[IBIS VER]   4.1
[File Name]   f29h85xpts.ibs
[File Rev]   1.0
[Date]   May 06, 2024
[Source]   File originated at Texas Instruments
[Copyright]   (c) 2012, Texas Instruments Inc.
[Component]   f29h85xpts
[Manufacturer]  Texas Instruments
[Package]
| Variable   Typ   Min   Max
R_pkg   2.65E-01   1.10E-01   3.57E-01
L_pkg   7.29E-09   5.43E-09   8.54E-09
C_pkg   1.07E-13   7.65E-14   2.05E-13
[Pin]   signal_name   model_name   R_pin   L_pin   C_pin
1   GPIO15   BQ33100HYPBFZ_PMB_5FS_LC_7LM   2.94E-01   8.32E-09   2.03E-13
2   GPIO16   BCF33100DSHYPBFZ_USF_7LM   2.97E-01   8.27E-09   1.00E-13
3   VDDIO   NC   2.90E-01   8.13E-09   9.86E-14
4   GPIO17   BCF33100DSHYPBFZ_USF_7LM   2.88E-01   8.03E-09   9.72E-14
5   GPIO19   BCF33100DSHYPBFZ_USF_7LM   2.82E-01   7.90E-09   9.58E-14
6   GPIO20   BCF33100DSHYPBFZ_USF_7LM   2.77E-01   7.78E-09   9.44E-14
7   GPIO21   BCF33100DSHYPBFZ_USF_7LM   2.72E-01   7.66E-09   9.30E-14
8   VDD   NC   1.59E-01   6.53E-09   9.39E-14
9   GPIO34   BCF33100DSHYPBFZ_USF_7LM   2.96E-01   7.73E-09   9.06E-14
10   GPIO35   BCF33100DSHYPBFZ_USF_7LM   2.90E-01   7.59E-09   8.92E-14
11   VDD   NC   1.75E-01   6.46E-09   9.05E-14
12   VDDIO   NC   3.57E-01   8.06E-09   8.71E-14
13   GPIO18   BQ33100HYPBFZ_PMB_5FS_LC_7LM   3.47E-01   7.89E-09   8.56E-14
14   GPIO22   BQ33100HYPBFZ_PMB_5FS_LC_7LM   3.44E-01   7.80E-09   8.43E-14
15   B11,GPIO235   BCF33100DSHYPBFZ_USF_7LM   3.42E-01   7.70E-09   8.29E-14
16   B10,GPIO234   BCF33100DSHYPBFZ_USF_7LM   3.33E-01   7.54E-09   8.15E-14
17   A11,GPIO229   BCF33100DSHYPBFZ_USF_7LM   3.24E-01   7.38E-09   8.01E-14
18   A10,GPIO228   BCF33100DSHYPBFZ_USF_7LM   3.16E-01   7.23E-09   7.86E-14
19   B9,GPIO233   BCF33100DSHYPBFZ_USF_7LM   3.08E-01   7.08E-09   7.72E-14
20   B8,GPIO232   BCF33100DSHYPBFZ_USF_7LM   3.01E-01   6.94E-09   2.04E-13
21   A9,GPIO227   BCF33100DSHYPBFZ_USF_7LM   2.95E-01   6.80E-09   2.00E-13
22   A8,GPIO226   BCF33100DSHYPBFZ_USF_7LM   2.89E-01   6.68E-09   1.96E-13
23   B7/E27,GPIO231   BCF33100DSHYPBFZ_USF_7LM   2.88E-01   6.66E-09   1.96E-13
24   B6/E26,GPIO230   BCF33100DSHYPBFZ_USF_7LM   2.82E-01   6.69E-09   2.00E-13
25   A7/E25,GPIO225   BCF33100DSHYPBFZ_USF_7LM   2.77E-01   6.72E-09   2.03E-13
26   A6/E24,GPIO224   BCF33100DSHYPBFZ_USF_7LM   2.73E-01   6.75E-09   7.69E-14
27   VDDA   NC   1.63E-01   5.81E-09   8.07E-14
28   VSSA   NC   1.61E-01   5.86E-09   8.20E-14
29   B5/D31   ICF33SHYPB_LC_7LM   2.81E-01   7.05E-09   8.10E-14
30   B4/D30   ICF33SHYPB_LC_7LM   2.74E-01   7.06E-09   8.23E-14
31   A5/D29   ICF33SHYPB_LC_7LM   2.68E-01   7.09E-09   8.36E-14
32   A4/D28   ICF33SHYPB_LC_7LM   2.63E-01   7.12E-09   8.49E-14
33   B3/D27   ICF33SHYPB_LC_7LM   2.60E-01   7.17E-09   8.62E-14
34   B2/D26   ICF33SHYPB_LC_7LM   2.58E-01   7.22E-09   8.75E-14
35   A3/D25   ICF33SHYPB_LC_7LM   2.57E-01   7.29E-09   8.89E-14
36   A2/D24   ICF33SHYPB_LC_7LM   2.58E-01   7.38E-09   9.02E-14
37   VREFLOAB   NC   1.51E-01   6.46E-09   9.36E-14
38   VREFHIAB   NC   1.15E-01   6.20E-09   9.70E-14
39   A15/B15/C15/D15/E15   ICF33SHYPB_LC_7LM   2.63E-01   7.65E-09   9.43E-14
40   A14/B14/C14/D14/E14   ICF33SHYPB_LC_7LM   2.67E-01   7.76E-09   9.57E-14
41   B1/C27   ICF33SHYPB_LC_7LM   2.73E-01   7.89E-09   9.71E-14
42   B0/C26/VDAC   ICF33SHYPB_LC_7LM   2.80E-01   8.03E-09   9.85E-14
43   A1/C25   ICF33SHYPB_LC_7LM   2.88E-01   8.19E-09   9.99E-14
44   A0/C24/DACA_OUT   ICF33SHYPB_LC_7LM   2.98E-01   8.36E-09   2.03E-13
45   C0/E28   ICF33SHYPB_LC_7LM   2.98E-01   8.43E-09   2.05E-13
46   C1/E29   ICF33SHYPB_LC_7LM   2.88E-01   8.26E-09   1.01E-13
47   D0/B24   ICF33SHYPB_LC_7LM   2.79E-01   8.10E-09   9.98E-14
48   D1/B25   ICF33SHYPB_LC_7LM   2.72E-01   7.96E-09   9.83E-14
49   E0/A24/DACC_OUT   ICF33SHYPB_LC_7LM   2.66E-01   7.82E-09   9.69E-14
50   E1/A25   ICF33SHYPB_LC_7LM   2.61E-01   7.70E-09   9.55E-14
51   C2/E30   ICF33SHYPB_LC_7LM   2.57E-01   7.59E-09   9.41E-14
52   C3/E31   ICF33SHYPB_LC_7LM   2.55E-01   7.49E-09   9.27E-14
53   VREFLOCDE   NC   1.48E-01   6.42E-09   9.33E-14
54   VREFHICDE   NC   1.10E-01   6.00E-09   9.39E-14
55   C4   ICF33SHYPB_LC_7LM   2.55E-01   7.26E-09   8.87E-14
56   C5   ICF33SHYPB_LC_7LM   2.57E-01   7.20E-09   8.73E-14
57   D2/B26   ICF33SHYPB_LC_7LM   2.60E-01   7.15E-09   8.60E-14
58   D3/B27   ICF33SHYPB_LC_7LM   2.65E-01   7.12E-09   8.47E-14
59   E2/A26   ICF33SHYPB_LC_7LM   2.70E-01   7.09E-09   8.33E-14
60   E3/A27   ICF33SHYPB_LC_7LM   2.77E-01   7.08E-09   8.20E-14
61   VSSA   NC   1.58E-01   5.90E-09   8.29E-14
62   VDDA   NC   1.60E-01   5.84E-09   8.17E-14
63   C6,GPIO236   BCF33100DSHYPBFZ_USF_7LM   2.73E-01   6.81E-09   7.79E-14
64   C7,GPIO237   BCF33100DSHYPBFZ_USF_7LM   2.70E-01   6.71E-09   7.65E-14
65   D4/B28,GPIO240   BCF33100DSHYPBFZ_USF_7LM   2.70E-01   6.63E-09   2.02E-13
66   D5/B29,GPIO241   BCF33100DSHYPBFZ_USF_7LM   2.68E-01   6.54E-09   1.99E-13
67   E4/A28,GPIO246   BCF33100DSHYPBFZ_USF_7LM   2.67E-01   6.52E-09   1.99E-13
68   E5/A29,GPIO247   BCF33100DSHYPBFZ_USF_7LM   2.66E-01   6.59E-09   2.02E-13
69   C8,GPIO238   BCF33100DSHYPBFZ_USF_7LM   2.66E-01   6.67E-09   7.65E-14
70   C9,GPIO239   BCF33100DSHYPBFZ_USF_7LM   2.67E-01   6.76E-09   7.79E-14
71   D6/B30,GPIO242   BCF33100DSHYPBFZ_USF_7LM   2.69E-01   6.85E-09   7.93E-14
72   D7/B31,GPIO243   BCF33100DSHYPBFZ_USF_7LM   2.72E-01   6.96E-09   8.06E-14
73   E6/A30,GPIO248   BCF33100DSHYPBFZ_USF_7LM   2.76E-01   7.07E-09   8.20E-14
74   E7/A31,GPIO249   BCF33100DSHYPBFZ_USF_7LM   2.81E-01   7.19E-09   8.34E-14
75   D8/C28,GPIO244   BCF33100DSHYPBFZ_USF_7LM   2.87E-01   7.32E-09   8.48E-14
76   D9/C29,GPIO245   BCF33100DSHYPBFZ_USF_7LM   2.93E-01   7.46E-09   8.63E-14
77   GPIO222/TDI   BCF33100DSHYPBFZ_USF_7LM   3.00E-01   7.60E-09   8.77E-14
78   GPIO223/TDO   BCPF335585DSHYPBFZ_USF_7LM   3.07E-01   7.75E-09   8.91E-14
79   VDDIO   NC   3.15E-01   7.89E-09   9.05E-14
80   VDD   NC   1.33E-01   6.28E-09   9.70E-14
81   VDD3VFL   NC   1.29E-01   6.32E-09   9.80E-14
82   TMS   BCF3355DSHYPBFZ_TMS_USF_7LM   3.07E-01   8.05E-09   9.46E-14
83   TCK   IQ0442FS_40P60P_3X2_USF_7LM   3.16E-01   8.21E-09   9.60E-14
84   VDD   NC   1.33E-01   6.59E-09   1.02E-13
85   GPIO37   BCF33100DSHYPBFZ_7LM   3.13E-01   8.34E-09   9.87E-14
86   GPIO39   BCF33100DSHYPBFZ_7LM   3.08E-01   8.37E-09   1.00E-13
87   GPIO40   BCF33100DSHYPBFZ_7LM   3.18E-01   8.54E-09   1.01E-13
88   VDDIO   NC   2.94E-01   8.39E-09   2.05E-13
89   GPIO41   BCF33100DSHYPBFZ_CORNER_USF_7LM   2.94E-01   8.32E-09   2.03E-13
90   GPIO48   BCF33100DSHYPBFZ_USF_7LM   2.92E-01   8.22E-09   9.99E-14
91   GPIO219/ERRORSTS   BCF33100DSHYPBFZ_CORNER_USF_7LM   2.96E-01   8.18E-09   9.86E-14
92   GPIO49   BCF33100DSHYPBFZ_USF_7LM   2.89E-01   8.05E-09   9.72E-14
93   GPIO50   BCF33100DSHYPBFZ_USF_7LM   2.83E-01   7.91E-09   9.58E-14
94   GPIO51   BCF33100DSHYPBFZ_USF_7LM   2.79E-01   7.79E-09   9.44E-14
95   GPIO52   BCF33100DSHYPBFZ_USF_7LM   2.78E-01   7.71E-09   9.31E-14
96   GPIO53   BCF33100DSHYPBFZ_USF_7LM   2.73E-01   7.59E-09   9.17E-14
97   GPIO54   BCF33100DSHYPBFZ_USF_7LM   2.70E-01   7.48E-09   9.03E-14
98   VDDIO   NC   2.67E-01   7.38E-09   8.90E-14
99   GPIO55   BCF33100DSHYPBFZ_USF_7LM   2.67E-01   7.31E-09   8.76E-14
100   GPIO56   BCF33100DSHYPBFZ_USF_7LM   2.65E-01   7.22E-09   8.63E-14
101   VDD3VFL   NC   1.15E-01   5.74E-09   8.92E-14
102   GPIO57   BCF33100DSHYPBFZ_USF_7LM   2.66E-01   7.07E-09   8.36E-14
103   GPIO58   BCF33100DSHYPBFZ_USF_7LM   2.66E-01   6.99E-09   8.22E-14
104   GPIO59   BCF3385DSHYPBFZ_USF_7LM   2.66E-01   6.92E-09   8.09E-14
105   VDD   NC   1.13E-01   5.43E-09   8.39E-14
106   GPIO60   BCF33100DSHYPBFZ_USF_7LM   2.67E-01   6.77E-09   7.82E-14
107   VDDIO   NC   2.69E-01   6.71E-09   7.69E-14
108   GPIO61   BCF33100DSHYPBFZ_USF_7LM   2.68E-01   6.63E-09   2.03E-13
109   GPIO62   BCF33100DSHYPBFZ_USF_7LM   2.69E-01   6.56E-09   2.00E-13
110   GPIO63   BCF33100DSHYPBFZ_USF_7LM   2.70E-01   6.50E-09   1.96E-13
111   GPIO64   BCF3385DSHYPBFZ_USF_7LM   2.72E-01   6.51E-09   1.96E-13
112   GPIO65   BCF33100DSHYPBFZ_USF_7LM   2.73E-01   6.60E-09   2.00E-13
113   GPIO66   BCF33100DSHYPBFZ_USF_7LM   2.73E-01   6.68E-09   2.03E-13
114   GPIO44   BCF33100DSHYPBFZ_USF_7LM   2.76E-01   6.78E-09   7.70E-14
115   VDDIO   NC   2.76E-01   6.86E-09   7.83E-14
116   GPIO45   BCF33100DSHYPBFZ_USF_7LM   2.77E-01   6.94E-09   7.96E-14
117   GPIO32   BCF33100DSHYPBFZ_USF_7LM   2.80E-01   7.05E-09   8.10E-14
118   GPIO127   BCF33100DSHYPBFZ_USF_7LM   2.81E-01   7.13E-09   8.24E-14
119   VDD   NC   1.17E-01   5.69E-09   8.81E-14
120   VDDOSC   NC   2.77E-01   7.25E-09   8.50E-14
121   GPIO221,X2   BCPF335585DSHYPBFZ_USF_7LM   2.71E-01   7.27E-09   8.63E-14
122   VSSOSC   NC   2.71E-01   7.34E-09   8.76E-14
123   GPIO220,X1   BCPF335585DSHYPBFZ_USF_7LM   2.74E-01   7.45E-09   8.90E-14
124   XRSn   BQ0491FS_3X2_USF_7LM   2.67E-01   7.46E-09   9.03E-14
125   GPIO38   BCF33100DSHYPBFZ_USF_7LM   2.70E-01   7.56E-09   9.17E-14
126   GPIO103   BCF33100DSHYPBFZ_USF_7LM   2.74E-01   7.67E-09   9.30E-14
127   VDDIO   NC   2.75E-01   7.76E-09   9.44E-14
128   GPIO46   BCF33100DSHYPBFZ_USF_7LM   2.75E-01   7.84E-09   9.57E-14
129   GPIO47   BCF33100DSHYPBFZ_USF_7LM   2.80E-01   7.96E-09   9.71E-14
130   GPIO42   BCPF335585DSHYPBFZ_USF_7LM   2.85E-01   8.08E-09   9.85E-14
131   GPIO43   BCF33100DSHYPBFZ_CORNER_USF_7LM   2.92E-01   8.22E-09   9.99E-14
132   GPIO67   BCF33100DSHYPBFZ_CORNER_USF_7LM   2.96E-01   8.33E-09   2.03E-13
133   GPIO68   BCF33100DSHYPBFZ_CORNER_USF_7LM   2.94E-01   8.39E-09   2.05E-13
134   GPIO69   BCF33100DSHYPBFZ_USF_7LM   2.91E-01   8.29E-09   1.01E-13
135   GPIO70   BCF3385DSHYPBFZ_CORNER_7LM   2.84E-01   8.14E-09   9.98E-14
136   GPIO71   BCF33100DSHYPBFZ_USF_7LM   2.78E-01   8.01E-09   9.84E-14
137   VDD   NC   1.62E-01   6.86E-09   9.92E-14
138   VDDIO   NC   2.87E-01   7.95E-09   9.57E-14
139   GPIO72   BCF33100DSHYPBFZ_USF_7LM   2.81E-01   7.81E-09   9.43E-14
140   GPIO73   BCF33100DSHYPBFZ_USF_7LM   2.76E-01   7.68E-09   9.29E-14
141   GPIO74   BCF33100DSHYPBFZ_USF_7LM   2.71E-01   7.56E-09   9.15E-14
142   GPIO75   BCF33100DSHYPBFZ_USF_7LM   2.70E-01   7.48E-09   9.02E-14
143   GPIO76   BCF33100DSHYPBFZ_USF_7LM   2.67E-01   7.37E-09   8.88E-14
144   GPIO77   BCF33100DSHYPBFZ_USF_7LM   2.64E-01   7.27E-09   8.74E-14
145   GPIO78   BCF33100DSHYPBFZ_USF_7LM   2.63E-01   7.18E-09   8.60E-14
146   GPIO79   BCF33100DSHYPBFZ_USF_7LM   2.62E-01   7.09E-09   8.46E-14
147   VDDIO   NC   2.63E-01   7.02E-09   8.33E-14
148   GPIO84   BCF33100DSHYPBFZ_USF_7LM   2.64E-01   6.96E-09   8.19E-14
149   GPIO31   BCF33100DSHYPBFZ_USF_7LM   2.67E-01   6.90E-09   8.06E-14
150   GPIO30   BCF3355DSHYPBFZ_USF_7LM   2.68E-01   6.84E-09   7.92E-14
151   GPIO29   BQ33100HYPBFZ_PMB_5FS_LC_7LM   2.70E-01   6.78E-09   7.79E-14
152   VDDIO   NC   2.69E-01   6.70E-09   7.65E-14
153   VDD   NC   1.52E-01   5.53E-09   2.04E-13
154   GPIO28   BCF33100DSHYPBFZ_USF_7LM   2.69E-01   6.54E-09   1.99E-13
155   GPIO27   BCF33100DSHYPBFZ_USF_7LM   2.68E-01   6.53E-09   1.99E-13
156   GPIO26   BCF33100DSHYPBFZ_USF_7LM   2.67E-01   6.60E-09   2.02E-13
157   GPIO25   BCF33100DSHYPBFZ_USF_7LM   2.66E-01   6.66E-09   7.65E-14
158   GPIO24   BCF33100DSHYPBFZ_USF_7LM   2.66E-01   6.74E-09   7.79E-14
159   GPIO23   BQ33100HYPBFZ_PMB_5FS_LC_7LM   2.67E-01   6.83E-09   7.92E-14
160   GPIO0   BCF33100DSHYPBFZ_USF_7LM   2.64E-01   6.88E-09   8.06E-14
161   GPIO1   BCF33100DSHYPBFZ_USF_7LM   2.65E-01   6.97E-09   8.19E-14
162   GPIO2   BCF33100DSHYPBFZ_USF_7LM   2.67E-01   7.06E-09   8.33E-14
163   GPIO3   BCF33100DSHYPBFZ_USF_7LM   2.70E-01   7.17E-09   8.47E-14
164   GPIO4   BCF33100DSHYPBFZ_USF_7LM   2.71E-01   7.25E-09   8.61E-14
165   GPIO5   BCF33100DSHYPBFZ_USF_7LM   2.74E-01   7.36E-09   8.75E-14
166   GPIO6   BCF3355DSHYPBFZ_USF_7LM   2.79E-01   7.48E-09   8.89E-14
167   GPIO7   BCF33100DSHYPBFZ_USF_7LM   2.81E-01   7.57E-09   9.02E-14
168   VDDIO   NC   2.82E-01   7.66E-09   9.16E-14
169   VDD   NC   1.70E-01   6.70E-09   9.55E-14
170   GPIO8   BCF33100DSHYPBFZ_USF_7LM   2.82E-01   7.82E-09   9.43E-14
171   GPIO9   BCF3385DSHYPBFZ_USF_7LM   2.89E-01   7.96E-09   9.58E-14
172   GPIO10   BQ33100HYPBFZ_PMB_5FS_LC_7LM   2.86E-01   8.01E-09   9.71E-14
173   GPIO11   BCF33100DSHYPBFZ_USF_7LM   2.87E-01   8.10E-09   9.85E-14
174   GPIO12   BCF33100DSHYPBFZ_CORNER_USF_7LM   2.89E-01   8.19E-09   9.98E-14
175   GPIO13   BCF33100DSHYPBFZ_USF_7LM   2.91E-01   8.29E-09   1.01E-13
176   GPIO14   BCF33100DSHYPBFZ_CORNER_USF_7LM   2.96E-01   8.41E-09   2.05E-13
| End of package information
|   Component BCF33100DSHYPBFZ_7LM
[Component]   BCF33100DSHYPBFZ_7LM
[Manufacturer]  IO Methodology Inc.
[Package]
|   typ   min   max
R_pkg   0   0   0
L_pkg   0   0   0
C_pkg   0   0   0
[Pin]   signal_name  model_name   R_pin   L_pin   C_pin
VSS   VSS   GND
VDDS   VDDS   POWER
PAD   PAD   BCF33100DSHYPBFZ_7LM
[Model Selector] BCF33100DSHYPBFZ_7LM
WK_PU_ON_3P3  Cell operated at 3.3(nom)
|WK_PU_ON_3P3; WEAK_PULLUP_ON
WK_PD_ON_3P3  Cell operated at 3.3(nom)
|WK_PD_ON_3P3; WEAK_PULLDOWN_ON
DRIVER_MODE_3P3  Cell operated at 3.3(nom)
|DRIVER_MODE_3P3
RECEIVER_MODE_3P3  Cell operated at 3.3(nom)
|   Component BCF33100DSHYPBFZ_USF_7LM
[Component]   BCF33100DSHYPBFZ_USF_7LM
[Manufacturer]  Texas Instruments
[Package]
| variable   typ   min   max
R_pkg   0.0   0.0   0.0
L_pkg   0.0H   0.0H   0.0H
C_pkg   0.0F   0.0F   0.0F
[Pin]  signal_name   model_name   R_pin   L_pin   C_pin
PAD   PAD   BCF33100_USF_7LM_IO_3.3V   0   0   0
VDDS   VDDS   Power   0   0   0
VSS   VSS   Gnd   0   0   0
[Model Selector] BCF33100DSHYPBFZ_USF_7LM
BCF33100_USF_7LM_IO_3.3V I/O model with 3.3V supply
|   Component BCF33100DSHYPBFZ_CORNER_USF_7LM
[Component]   BCF33100DSHYPBFZ_CORNER_USF_7LM
[Manufacturer]  Texas Instruments
[Package]
| variable   typ   min   max
R_pkg   0.0   0.0   0.0
L_pkg   0.0H   0.0H   0.0H
C_pkg   0.0F   0.0F   0.0F
[Pin]  signal_name   model_name   R_pin   L_pin   C_pin
PAD   PAD   BCF33100_CORNER_7LM_IO_3.3V   0   0   0
VDDS   VDDS   Power   0   0   0
VSS   VSS   Gnd   0   0   0
[Model Selector] BCF33100DSHYPBFZ_CORNER_USF_7LM
BCF33100_CORNER_7LM_IO_3.3V  I/O model with 3.3V supply
|   Component BCF3355DSHYPBFZ_TMS_USF_7LM
[Component]   BCF3355DSHYPBFZ_TMS_USF_7LM
[Manufacturer]  Texas Instruments
[Package]
| variable   typ   min   max
R_pkg   0.0   0.0   0.0
L_pkg   0.0H   0.0H   0.0H
C_pkg   0.0F   0.0F   0.0F
[Pin]  signal_name   model_name   R_pin   L_pin   C_pin
PAD   PAD   BCF3355_TMS_7LM_IO_3.3V   0   0   0
VDDS   VDDS   Power   0   0   0
VSS   VSS   Gnd   0   0   0
[Model Selector] BCF3355DSHYPBFZ_TMS_USF_7LM
BCF3355_TMS_7LM_IO_3.3V I/O model with 3.3V supply
|   Component IQ0442FS_40P60P_3X2_USF_7LM
[Component]   IQ0442FS_40P60P_3X2_USF_7LM
[Manufacturer]  Texas Instruments
[Package]
| variable   typ   min   max
R_pkg   0.0   0.0   0.0
L_pkg   0.0H   0.0H   0.0H
C_pkg   0.0F   0.0F   0.0F
[Pin]  signal_name   model_name   R_pin   L_pin   C_pin
PAD   PAD   IQRX_3.3V   0   0   0
VDDS   VDDS   Power   0   0   0
VSS   VSS   Gnd   0   0   0
[Model Selector] IQ0442FS_40P60P_3X2_USF_7LM
IQRX_3.3V I/O model with 3.3V supply
|   Component BCF3355DSHYPBFZ_USF_7LM
[Component]   BCF3355DSHYPBFZ_USF_7LM
[Manufacturer]  Texas Instruments
[Package]
| variable   typ   min   max
R_pkg   0.0   0.0   0.0
L_pkg   0.0H   0.0H   0.0H
C_pkg   0.0F   0.0F   0.0F
[Pin]  signal_name   model_name   R_pin   L_pin   C_pin
PAD   PAD   BCF3355_USF_7LM_IO_3.3V   0   0   0
VDDS   VDDS   Power   0   0   0
VSS   VSS   Gnd   0   0   0
[Model Selector] BCF3355DSHYPBFZ_USF_7LM
BCF3355_USF_7LM_IO_3.3V I/O model with 3.3V supply
|   Component BCF3385DSHYPBFZ_CORNER_7LM
[Component]   BCF3385DSHYPBFZ_CORNER_7LM
[Manufacturer]  IO Methodology Inc.
[Package]
|   typ   min   max
R_pkg   0   0   0
L_pkg   0   0   0
C_pkg   0   0   0
[Pin]   signal_name  model_name   R_pin   L_pin   C_pin
VSS   VSS   GND
VDDS   VDDS   POWER
PAD   PAD   BCF3385DSHYPBFZ_CORNER_7LM
[Model Selector] BCF3385DSHYPBFZ_CORNER_7LM
WK_PU_ON_3P3_BCF3385DSHYPBFZ_CORNER_7LM  Cell operated at 3.3(nom)
|WK_PU_ON_3P3; WEAK_PULLUP_ON
WK_PD_ON_3P3_BCF3385DSHYPBFZ_CORNER_7LM  Cell operated at 3.3(nom)
|WK_PD_ON_3P3; WEAK_PULLDOWN_ON
DRIVER_MODE_3P3_BCF3385_CORNER_7LM Cell operated at 3.3(nom)
|DRIVER_MODE_3P3
RECEIVER_MODE_3P3_BCF3385_CORNER_7LM  Cell operated at 3.3(nom)
|   Component BCF3385DSHYPBFZ_USF_7LM
[Component]   BCF3385DSHYPBFZ_USF_7LM
[Manufacturer]  Texas Instruments
[Package]
| variable   typ   min   max
R_pkg   0.0   0.0   0.0
L_pkg   0.0H   0.0H   0.0H
C_pkg   0.0F   0.0F   0.0F
[Pin]  signal_name   model_name   R_pin   L_pin   C_pin
PAD   PAD   BCF3385_USF_7LM_IO_3.3V   0   0   0
VDDS   VDDS   Power   0   0   0
VSS   VSS   Gnd   0   0   0
[Model Selector] BCF3385DSHYPBFZ_USF_7LM
BCF3385_USF_7LM_IO_3.3V I/O model with 3.3V supply
|   Component BCPF335585DSHYPBFZ_USF_7LM
[Component]   BCPF335585DSHYPBFZ_USF_7LM
[Manufacturer]  Texas Instruments
[Package]
| variable   typ   min   max
R_pkg   0.0   0.0   0.0
L_pkg   0.0H   0.0H   0.0H
C_pkg   0.0F   0.0F   0.0F
[Pin]  signal_name   model_name   R_pin   L_pin   C_pin
PAD   PAD   BCPF335585DSHYPBFZ_USF_7LM   0   0   0
VDDS   VDDS   Power   0   0   0
VSS   VSS   Gnd   0   0   0
[Model Selector]   BCPF335585DSHYPBFZ_USF_7LM
BCPF335585_7LM_IO_DS0_3.3V   I/O model DS 0 with 3.3V supply
BCPF335585_7LM_IO_DS1_3.3V   I/O model DS 1 with 3.3V supply
|   Component BQ0491FS_3X2_USF_7LM
[Component]   BQ0491FS_3X2_USF_7LM
[Manufacturer]  Texas Instruments
[Package]
| variable   typ   min   max
R_pkg   0.0   0.0   0.0
L_pkg   0.0H   0.0H   0.0H
C_pkg   0.0F   0.0F   0.0F
[Pin]  signal_name   model_name   R_pin   L_pin   C_pin
PAD   PAD   BQ0491FS_3X2_USF_7LM   0   0   0
VDDS   VDDS   Power   0   0   0
VSS   VSS   Gnd   0   0   0
[Model Selector]   BQ0491FS_3X2_USF_7LM
BQ0491_3X2_USF_7LM_IO_15p_3p3   I/O open drain model with C_fixture 15pF for 3.3V supply
BQ0491_3X2_USF_7LM_IO_50p_3p3   I/O open drain model with C_fixture 50pF for 3.3V supply
BQ0491_3X2_USF_7LM_IO_100p_3p3   I/O open drain model with C_fixture 100pF for 3.3V supply
BQ0491_3X2_USF_7LM_IO_150p_3p3   I/O open drain model with C_fixture 150pF for 3.3V supply
|   Component BQ33100HYPBFZ_PMB_5FS_LC_7LM
[Component]   BQ33100HYPBFZ_PMB_5FS_LC
[Manufacturer]  Texas Instruments
[Package]
| variable   typ   min   max
R_pkg   0.0   0.0   0.0
L_pkg   0.0H   0.0H   0.0H
C_pkg   0.0F   0.0F   0.0F
[Pin]  signal_name   model_name   R_pin   L_pin   C_pin
Pin1   PAD   BQ33100HYPBFZ_PMB_5FS_LC_7LM   0   0   0
Pin2   VDDS   Power   0   0   0
Pin3   VSS   Gnd   0   0   0
[Model Selector]   BQ33100HYPBFZ_PMB_5FS_LC_7LM
BQ33_PMB_IO_M0_D0   I/O model with Mode = 0 and Drive = 0
BQ33_PMB_IO_M0_D1   I/O model with Mode = 0 and Drive = 1
BQ33_PMB_IO_M1_D0   I/O model with Mode = 1 and Drive = 0
BQ33_PMB_IO_M1_D1   I/O model with Mode = 1 and Drive = 1
|   Component IQ0440FS_VREGENZ_PU_7LM
[Component]   IQ0440FS_VREGENZ_PU_7LM
[Manufacturer]  Texas Instruments
[Package]
|   typ   min   max
R_pkg   0   0   0
L_pkg   0   0   0
C_pkg   0   0   0
[Pin]   signal_name  model_name   R_pin   L_pin   C_pin
VSS   VSS   GND
VDDS   VDDS   POWER
PAD   PAD   IQ0440FS_VREGENZ_PU_7LM
[Model Selector] IQ0440FS_VREGENZ_PU_7LM
WK_PD_ON_3P3_IQ0440FS_VREGENZ_PU_7LM Cell operated at 3.3(nom)
|WK_PD_ON_3P3; WEAK_PULLDOWN_ON
RECEIVER_MODE_3P3_IQ0440FS_VREGENZ  Cell operated at 3.3(nom)
|   Component ICF33SHYPB_LC_7LM
[Component]   ICF33SHYPB_LC_7LM
[Manufacturer]   Texas Instruments
[Package]
|  variable   typ   min   max
R_pkg   0   0   0
L_pkg   0   0   0
C_pkg   0   0   0
[Pin]   signal_name   model_name   R_pin   L_pin   C_pin
VSS   VSS   GND
VDDS   VDDS   POWER
PAD   PAD   ICF33SHYPB_LC_7LM
[Model Selector] ICF33SHYPB_LC_7LM
RECEIVER_MODE_3P3_ICF_7LM  Cell operated at 3.3(nom)
|RECEIVER_MODE_3P3_ICF_7LM; RECEIVER_MODE
WK_PU_ON_3P3_ICF_7LM  Cell operated at 3.3(nom)
|WK_PU_ON_3P3_ICF_7LM; WEAK_PULLUP_ON
WK_PD_ON_3P3_ICF_7LM  Cell operated at 3.3(nom)
| Models and submodels in the file (29): WK_PU_ON_3P3 (Input), WK_PD_ON_3P3 (Input), DRIVER_MODE_3P3 (I/O), RECEIVER_MODE_3P3 (Input), BCF33100_USF_7LM_IO_3.3V (I/O), BCF33100_CORNER_7LM_IO_3.3V (I/O), BCF3355_TMS_7LM_IO_3.3V (I/O), IQRX_3.3V (Input), BCF3355_USF_7LM_IO_3.3V (I/O), WK_PU_ON_3P3_BCF3385DSHYPBFZ_CORNER_7LM (Input), WK_PD_ON_3P3_BCF3385DSHYPBFZ_CORNER_7LM (Input), DRIVER_MODE_3P3_BCF3385_CORNER_7LM (I/O), RECEIVER_MODE_3P3_BCF3385_CORNER_7LM (Input), BCF3385_USF_7LM_IO_3.3V (I/O), BCPF335585_7LM_IO_DS0_3.3V (I/O), BCPF335585_7LM_IO_DS1_3.3V (I/O), BQ0491_3X2_USF_7LM_IO_15p_3p3 (I/O_open_drain), BQ0491_3X2_USF_7LM_IO_50p_3p3 (I/O_open_drain), BQ0491_3X2_USF_7LM_IO_100p_3p3 (I/O_open_drain), BQ0491_3X2_USF_7LM_IO_150p_3p3 (I/O_open_drain), BQ33_PMB_IO_M0_D0 (I/O), BQ33_PMB_IO_M0_D1 (I/O), BQ33_PMB_IO_M1_D0 (I/O), BQ33_PMB_IO_M1_D1 (I/O), WK_PD_ON_3P3_IQ0440FS_VREGENZ_PU_7LM (Input), RECEIVER_MODE_3P3_IQ0440FS_VREGENZ (Input), RECEIVER_MODE_3P3_ICF_7LM (Input), WK_PU_ON_3P3_ICF_7LM (Input), WK_PD_ON_3P3_ICF_7LM (Input)
